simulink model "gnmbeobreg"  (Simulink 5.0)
settings: Solver=ode45  StartTime=0.0  StopTime=Tstop  MaxStep=step_max  RelTol=1e-3
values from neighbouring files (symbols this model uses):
  beob = estim(sys,l,1,1)    [gnmbeobl_i.m]    (also in gnmbeobregl_i.m = estim(sysbeob,l,1,1); gnmbeobregs_i.m = ss(beob.a,beob.b,beob.c,beob.d); gnmbeobreg_i.m = ss([],[0 0],[],0); gnmbeobs_i.m = ss(beob.a,beob.b,beob.c,beob.d))
  CE = 2*pi*CM    (= 240.017678734)    [gnm_i.m]
  CM = 38.2    [gnm_i.m]
  J = 0.012    [gnm_i.m]
  k = place(syszreg.a,syszreg.b,polc)    [gnmbeobregl_i.m]    (also in gnmbeobregs_i.m; gnmbeobreg_i.m = [ 0 0 0 ])
  K_V = -1/(syszreg.c*inv(syszreg.a-syszreg.b*k)*syszreg.b)    [gnmbeobregl_i.m]    (also in gnmbeobregs_i.m; gnmbeobreg_i.m = 1)
  MW = 10    [gnmbeobreg_i.m]    (also in gnmbeob_i.m; gnmregn_i.m = 100; gnm_i.m = 0; lsg_gnmregnss_ini.m = 100)
  N_soll = 500/60    (= 8.33333333333)    [gnmbeobreg_i.m]    (also in gnmregn_i.m; lsg_gnmregnss_ini.m)
  PsiN = 0.04    [gnm_i.m]
  RA = 0.250    (= 0.25)    [gnm_i.m]
  T_MW = 0.4    [gnmbeobreg_i.m]    (also in gnmbeob_i.m; gnmregn_i.m = 0.1; gnm_i.m = 0; lsg_gnmregnss_ini.m = 0.1)
  T_Nsoll = 0.8    [gnmbeobreg_i.m]    (also in gnmregn_i.m = 0.4; lsg_gnmregnss_ini.m = 0.4)
  T_t = 0.0001    [gnmbeobreg_i.m]    (also in gnmbeob_i.m; gnmregi_i.m)
  TA = LA / RA    (= 0.016)    [gnm_i.m]
libraries: simulink x1

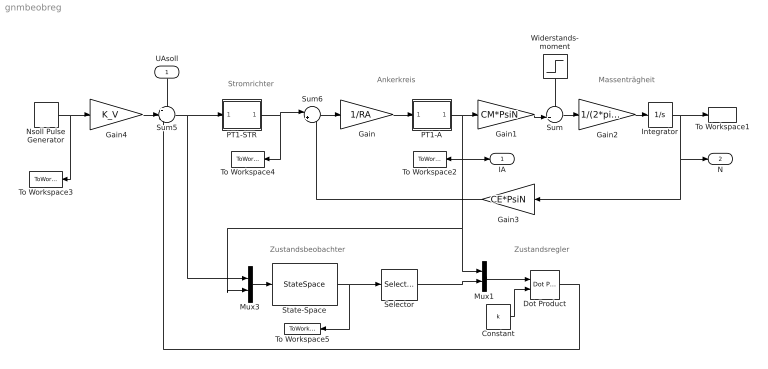
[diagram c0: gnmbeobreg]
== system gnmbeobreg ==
  note: Massenträgheit
  note: Ankerkreis
  note: Stromrichter
  note: Zustandsbeobachter
  note: Zustandsregler
  UAsoll : Inport  Orientation=down  PortDimensions=1
  Constant : Constant  Value=k
  Dot Product : simulink/Math Operations/Dot Product
  Gain : Gain  Gain=1/RA
  Gain1 : Gain  Gain=CM*PsiN
  Gain2 : Gain  Gain=1/(2*pi*J)
  Gain3 : Gain  Orientation=left  Gain=CE*PsiN
  Gain4 : Gain  Gain=K_V
  Integrator : Integrator
  Mux1 : Mux  Inputs=2
  Mux3 : Mux  Inputs=2
  Nsoll Pulse Generator : DiscretePulseGenerator  PulseType=Time based  Amplitude=N_soll  Period=T_Nsoll  PulseWidth=50
  PT1-A : Subsystem  mask(PT1){T=TA}
      mask prompts: T "Zeitkonstante"
      mask help: PT1 mit rückgekoppeltem Integrierer
  PT1-STR : Subsystem  mask(PT1){T=T_t}
      mask prompts: T "Zeitkonstante"
      mask help: PT1 mit rückgekoppeltem Integrierer
  Selector : Selector  Elements=sel_aus  InputPortWidth=sel_in
  State-Space : StateSpace  A=beob.a  B=beob.b  C=beob.c  D=beob.d  X0=0 %beobx0
  Sum : Sum  Inputs=-+|
  Sum5 : Sum  Inputs=++-
  Sum6 : Sum  Inputs=|+-
  To Workspace1 : ToWorkspace  VariableName=N  SampleTime=-1  SaveFormat=Array
  To Workspace2 : ToWorkspace  VariableName=IA  SampleTime=-1  SaveFormat=Array
  To Workspace3 : ToWorkspace  VariableName=Nsoll  SampleTime=-1  SaveFormat=Array
  To Workspace4 : ToWorkspace  VariableName=UA  SampleTime=-1  SaveFormat=Array
  To Workspace5 : ToWorkspace  VariableName=ybeob  SampleTime=-1  SaveFormat=Array
  Widerstands- moment : Step  Orientation=down  Time=T_MW  After=MW  SampleTime=0
  IA : Outport
  N : Outport  Port=2
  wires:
  Gain/1 -> PT1-A/1(In1)
  Gain1/1 -> Sum/2
  Widerstands- moment/1 -> Sum/1
  Sum/1 -> Gain2/1
  Gain2/1 -> Integrator/1
  Integrator/1 -> To Workspace1/1, N/1, Gain3/1
  Gain3/1 -> Sum6/2
  PT1-A/1(Out1) -> Gain1/1, To Workspace2/1, IA/1, Mux3/2, Mux1/1
  Sum6/1 -> Gain/1
  PT1-STR/1(Out1) -> Sum6/1, To Workspace4/1
  Nsoll Pulse Generator/1 -> To Workspace3/1, Gain4/1
  UAsoll/1 -> Sum5/1
  Gain4/1 -> Sum5/2
  Sum5/1 -> PT1-STR/1(In1), Mux3/1
  Mux3/1 -> State-Space/1
  State-Space/1 -> To Workspace5/1, Selector/1
  Constant/1 -> Dot Product/2
  Mux1/1 -> Dot Product/1
  Selector/1 -> Mux1/2
  Dot Product/1 -> Sum5/3

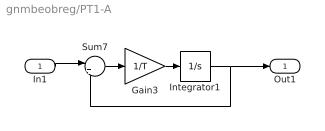
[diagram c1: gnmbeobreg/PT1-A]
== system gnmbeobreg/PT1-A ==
  In1 : Inport
  Gain3 : Gain  Gain=1/T
  Integrator1 : Integrator
  Sum7 : Sum  Inputs=|+-
  Out1 : Outport
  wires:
  Integrator1/1 -> Sum7/2, Out1/1
  Gain3/1 -> Integrator1/1
  Sum7/1 -> Gain3/1
  In1/1 -> Sum7/1

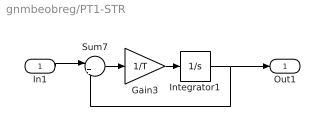
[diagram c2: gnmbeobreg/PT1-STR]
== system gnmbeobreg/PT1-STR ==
  In1 : Inport
  Gain3 : Gain  Gain=1/T
  Integrator1 : Integrator
  Sum7 : Sum  Inputs=|+-
  Out1 : Outport
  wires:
  Integrator1/1 -> Sum7/2, Out1/1
  Gain3/1 -> Integrator1/1
  Sum7/1 -> Gain3/1
  In1/1 -> Sum7/1
